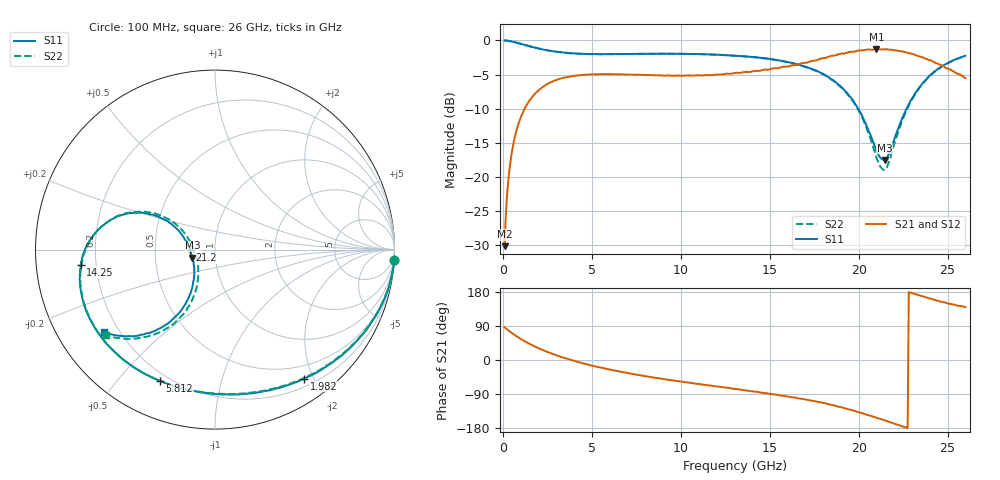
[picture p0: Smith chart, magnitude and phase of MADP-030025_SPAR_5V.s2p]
!Mean
# HZ S DB R 50
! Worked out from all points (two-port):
!   400 points, 100 MHz to 26 GHz, reference 50 ohm
!   highest |S21| = -1.27 dB at 21 GHz (marker M1); lowest = -30.1 dB at 100 MHz (marker M2)
!   |S21| within 3 dB of the highest: 14.73 GHz to 14.81 GHz (88.61 MHz wide, 0.6 % of centre); 14.94 GHz to 25.18 GHz (10.24 GHz wide, 51.1 % of centre)
!   lowest |S11| = -17.5 dB at 21.46 GHz (marker M3), VSWR 1.31, Z = 38.7 - j3.51 ohm
!   |S11| at or under -10 dB: 19.98 GHz to 22.69 GHz (2.714 GHz wide, 12.7 % of centre)
!   |S22| runs from -19.0 to 0.0 dB; largest |S21 - S12| = 0.0079
!   S11 on the Smith chart (normalised r, x): 100 MHz: 0, -34; 1.982 GHz: 0.31, -1.87; 5.812 GHz: 0.16, -0.65; 14.25 GHz: 0.14, -0.05; 21.2 GHz: 0.75, -0.00; 26 GHz: 0.14, -0.33
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1e8  -0.00 -3.4  -30.11 86.0  -30.11 86.1  -0.00 -3.2
1.6491e8  -0.01 -5.5  -25.77 83.5  -25.80 83.5  -0.01 -5.3
2.9474e8  -0.05 -9.7  -20.85 78.7  -20.84 78.8  -0.05 -9.5
6.193e8  -0.22 -20.0  -14.80 67.4  -14.81 67.4  -0.23 -19.5
1.1386e9  -0.59 -34.8  -10.46 51.8  -10.46 51.8  -0.59 -34.0
1.9825e9  -1.17 -55.3  -7.35 31.7  -7.34 31.7  -1.16 -53.9
3.1509e9  -1.70 -77.7  -5.66 10.2  -5.66 10.2  -1.71 -75.9
4.4491e9  -1.95 -96.9  -5.05 -8.1  -5.05 -8.0  -1.96 -95.0
5.8123e9  -2.00 -112.8  -4.94 -23.4  -4.94 -23.4  -2.01 -111.0
8.7982e9  -1.93 -138.8  -5.08 -48.4  -5.09 -48.5  -1.95 -137.4
1.3082e10  -2.22 -166.7  -4.75 -76.3  -4.77 -76.4  -2.23 -166.0
1.4251e10  -2.47 -173.7  -4.44 -83.7  -4.49 -83.8  -2.48 -173.2
1.7367e10  -4.17 165.7  -3.00 -107.2  -3.01 -107.0  -4.20 165.5
1.9639e10  -8.62 149.8  -1.64 -132.4  -1.69 -132.6  -8.74 148.0
2.1002e10  -16.18 168.4  -1.27 -152.4  -1.26 -152.3  -17.16 164.5
2.1196e10  -17.07 -179.5  -1.29 -155.2  -1.29 -155.2  -18.40 178.0
2.1456e10  -17.48 -160.5  -1.31 -159.1  -1.31 -159.1  -18.95 -159.3
2.1716e10  -16.55 -141.5  -1.33 -163.4  -1.34 -163.3  -17.70 -136.4
2.243e10  -11.48 -120.0  -1.59 -174.8  -1.59 -174.6  -11.80 -115.1
2.3404e10  -6.89 -121.2  -2.31 170.5  -2.29 170.4  -7.00 -118.1
2.4572e10  -3.98 -131.3  -3.52 154.2  -3.52 154.7  -4.04 -129.1
2.6e10  -2.24 -143.3  -5.52 139.2  -5.42 139.3  -2.26 -141.7
